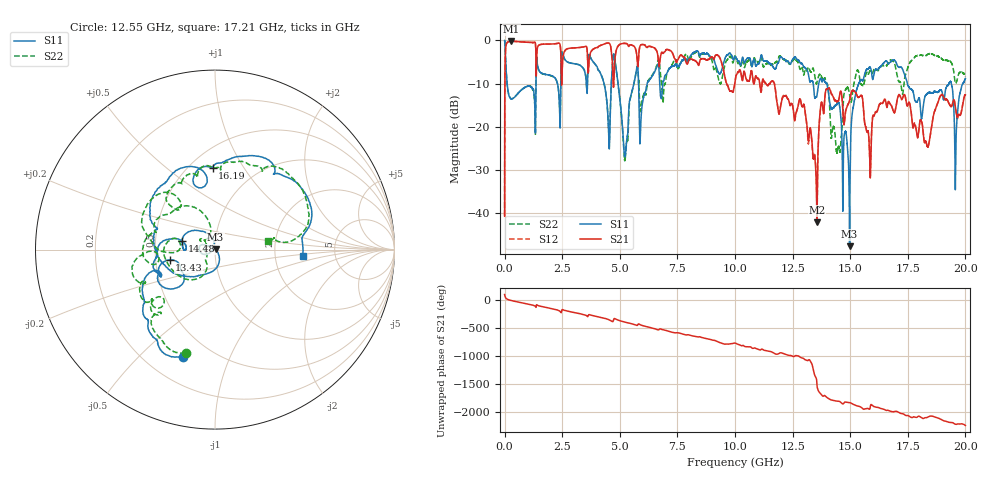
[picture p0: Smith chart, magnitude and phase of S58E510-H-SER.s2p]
!{S58E510}
!Johanson Technology Inc.
!www.johansontechnology.com
!Test Board Conditions:
!Substrate Type  RO4350B
!Substrate Thickness  60 mil
!Substrate Dk  3.66
!TL Type: GCPW
!TL Trace Width  115 mil
!TL Gap  52 mil
!Electrode orientation  Horizontal
!DUT TOPOLOGY	SERIES
!Mounting Pad LxW  55x428 mil
! Created Wed Apr 14 11:54:42 2021
# mhz S ma R 50
! 2 Port Network Data from SP1.SP block
! freq  magS11  angS11  magS21  angS21  magS12  angS12  magS22  angS22
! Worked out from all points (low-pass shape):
!   20001 points, 300 kHz to 20 GHz, reference 50 ohm
!   highest |S21| = -0.20 dB at 293.3 MHz (marker M1); lowest = -42.1 dB at 13.55 GHz (marker M2)
!   |S21| within 3 dB of the highest: 31.41 MHz to 1.358 GHz (1.326 GHz wide, 191 % of centre); 1.397 GHz to 2.441 GHz (1.045 GHz wide, 54.4 % of centre)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
!   lowest |S11| = -47.6 dB at 14.97 GHz (marker M3), VSWR 1.01, Z = 50.3 + j0.299 ohm
!   |S11| at or under -10 dB: 108.7 MHz to 1.357 GHz (1.248 GHz wide, 170 % of centre); 13.99 GHz to 15.37 GHz (1.384 GHz wide, 9.43 % of centre); 17.48 GHz to 19.29 GHz (1.802 GHz wide, 9.8 % of centre)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
!   |S22| runs from -27.8 to 0.0 dB; largest |S21 - S12| = 0.0096
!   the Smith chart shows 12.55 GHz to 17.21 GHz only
!   S11 on the Smith chart (normalised r, x): 12.55 GHz: 0.35, -0.68; 13.43 GHz: 0.59, -0.07; 14.48 GHz: 0.69, +0.07; 16.19 GHz: 0.64, +0.74; 17.21 GHz: 2.89, -0.29
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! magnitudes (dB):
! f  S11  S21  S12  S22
! 300 kHz  -0.1  -40.7  -40.6  -0.1
! 106.3 MHz  -9.9  -0.5  -0.5  -9.8
! 293.3 MHz  -13.5  -0.2  -0.2  -13.5
! 3.334 GHz  -6.0  -1.6  -1.6  -6.0
! 4.51 GHz  -20.6  -0.6  -0.6  -20.1
! 4.782 GHz  -4.2  -4.9  -4.8  -4.2
! 5.25 GHz  -25.9  -0.7  -0.7  -26.2
! 5.7 GHz  -7.5  -2.2  -2.2  -7.6
! 6.667 GHz  -5.5  -4.2  -4.2  -4.5
! 10 GHz  -3.8  -9.6  -9.7  -3.6
! 12.55 GHz  -4.1  -16.7  -16.7  -4.4
! 13.33 GHz  -9.4  -23.0  -23.4  -7.1
! 13.43 GHz  -11.7  -26.9  -26.5  -7.2
! 13.55 GHz  -12.8  -42.1  -40.5  -9.8
! 14.48 GHz  -14.5  -14.0  -14.1  -24.7
! 14.97 GHz  -47.6  -13.9  -14.0  -12.6
! 15.31 GHz  -10.9  -12.9  -12.9  -6.9
! 16.19 GHz  -6.8  -16.2  -16.1  -6.9
! 16.67 GHz  -5.5  -14.2  -14.1  -4.9
! 17.21 GHz  -6.2  -13.5  -13.6  -10.5
! 19.59 GHz  -23.5  -16.3  -16.4  -9.9
! 20 GHz  -8.8  -12.6  -12.5  -8.4
